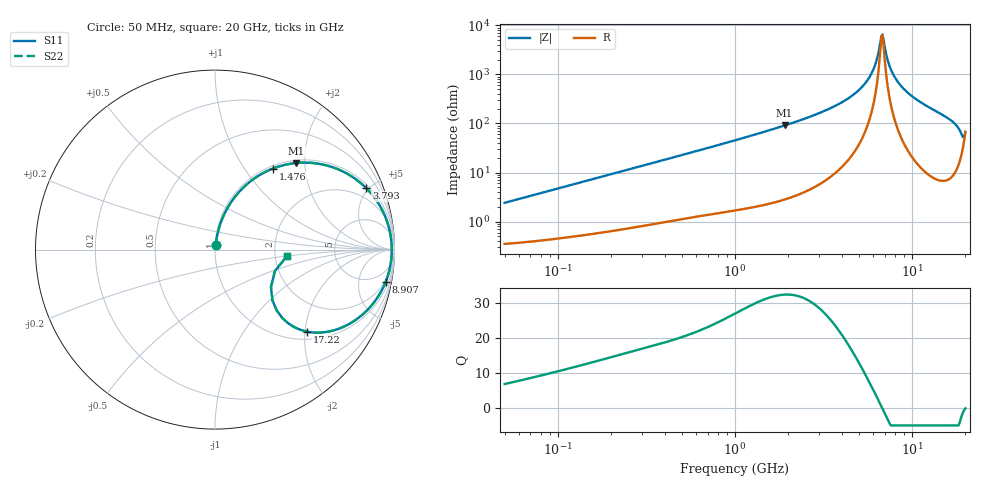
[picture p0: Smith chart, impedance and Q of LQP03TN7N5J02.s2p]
!Murata Part Number: LQP03TN7N5J02
!These Parameters are Measured in Series Mode Connection
!  o--[Z]--o
!Port1  Port2
!  o-------o
!Freq. Start=50[MHz] Stop=20[GHz], 401[Steps]
# Hz S RI R 50
!Freq.(Hz) S11(Real) S11(Imag) S21(Real) S21(Imag) S12(Real) S12(Imag) S22(Real) S22(Imag)
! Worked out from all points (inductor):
!   401 points, 50 MHz to 20 GHz, reference 50 ohm
!   read as one part in series: L = 7.56 nH near 51.52 MHz
!   highest Q = 32.3 at 1.904 GHz (marker M1), where L = 7.59 nH
!   self-resonance near 6.701 GHz
!   S11 on the Smith chart (normalised r, x): 50 MHz: 1.01, +0.05; 1.476 GHz: 1.04, +1.36; 3.793 GHz: 1.21, +4.82; 8.907 GHz: 2, -10; 17.22 GHz: 1.18, -2.05; 20 GHz: 2.34, -0.19
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5e7  0.00406 0.0237  0.9959 -0.0237  0.9959 -0.0237  0.00406 0.0237
1.364002e8  0.00916 0.0627  0.9908 -0.0627  0.9908 -0.0627  0.00916 0.0627
3.721004e8  0.0363 0.1615  0.9637 -0.1615  0.9637 -0.1615  0.0363 0.1615
1e9  0.179 0.3652  0.821 -0.3652  0.821 -0.3652  0.179 0.3652
1.476162e9  0.3231 0.4518  0.6769 -0.4518  0.6769 -0.4518  0.3231 0.4518
1.904239e9  0.4534 0.4826  0.5466 -0.4826  0.5466 -0.4826  0.4534 0.4826
2.728004e9  0.6651 0.4556  0.3349 -0.4556  0.3349 -0.4556  0.6651 0.4556
3.792786e9  0.8424 0.3428  0.1576 -0.3428  0.1576 -0.3428  0.8424 0.3428
4.748272e9  0.9293 0.225  0.0707 -0.225  0.0707 -0.225  0.9293 0.225
5.598765e9  0.9686 0.1245  0.0314 -0.1245  0.0314 -0.1245  0.9686 0.1245
6.125241e9  0.9803 0.0666  0.0197 -0.0666  0.0197 -0.0666  0.9803 0.0666
6.701223e9  0.985 0.00739  0.015 -0.00739  0.015 -0.00739  0.985 0.00739
6.905011e9  0.9849 -0.0125  0.0151 0.0125  0.0151 0.0125  0.9849 -0.0125
7.442007e9  0.9812 -0.0622  0.0188 0.0622  0.0188 0.0622  0.9812 -0.0622
8.020766e9  0.9722 -0.1116  0.0278 0.1116  0.0278 0.1116  0.9722 -0.1116
8.907419e9  0.9509 -0.1796  0.0491 0.1796  0.0491 0.1796  0.9509 -0.1796
1.050288e10  0.896 -0.2804  0.104 0.2804  0.104 0.2804  0.896 -0.2804
1.314879e10  0.7759 -0.3971  0.2241 0.3971  0.2241 0.3971  0.7759 -0.3971
1.721783e10  0.5135 -0.4572  0.4865 0.4572  0.4865 0.4572  0.5135 -0.4572
1.855685e10  0.3745 -0.3804  0.6255 0.3804  0.6255 0.3804  0.3745 -0.3804
1.912117e10  0.3203 -0.2834  0.6797 0.2834  0.6797 0.2834  0.3203 -0.2834
2e10  0.4032 -0.0337  0.5968 0.0337  0.5968 0.0337  0.4032 -0.0337
